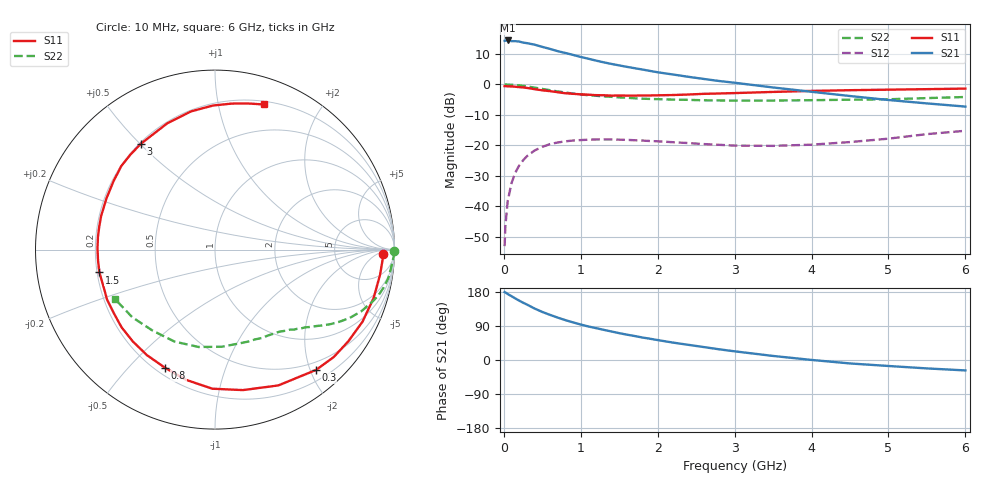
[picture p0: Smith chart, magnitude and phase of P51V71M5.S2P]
! SIEMENS Small Signal Semiconductors
! BFP183
! Si NPN RF Bipolar Junction Transistor in SOT143
! VCE = 1.75 V  IC = 1.5 mA
! Common Emitter S-Parameters:  March  1996
# GHz  S  MA  R  50
!  f  S11  S21  S12  S22
! GHz  MAG  ANG  MAG  ANG  MAG  ANG  MAG  ANG
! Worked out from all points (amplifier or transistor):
!   36 points, 10 MHz to 6 GHz, reference 50 ohm
!   highest |S21| = 14.4 dB at 50 MHz (marker M1)
!   |S21| within 3 dB of that: start of sweep to 630 MHz
!   unconditionally stable (mu >= 1): 2.223 GHz to end of sweep
!   at 250 MHz: K = 0.11, MSG = 19.3 dB, |S12| = -24.9 dB
!   at 1.4 GHz: K = 0.61, MSG = 12.4 dB, |S12| = -18.1 dB
!   at 6 GHz: K = 1.02, MAG = 3.2 dB, |S12| = -15.2 dB
!   S11 on the Smith chart (normalised r, x): 10 MHz: 26, -11; 300 MHz: 0.36, -2.09; 800 MHz: 0.24, -0.64; 1.5 GHz: 0.21, -0.09; 3 GHz: 0.21, +0.50; 6 GHz: 0.23, +1.37
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0.01  0.9373 -1.6  5.195 179.2  0.0022 83.9  0.9994 -0.6
0.02  0.9353 -3.5  5.226 178.3  0.0047 83.9  0.9991 -1.3
0.05  0.9302 -8.8  5.268 174.1  0.0121 86.5  0.993 -3.2
0.1  0.9238 -17.1  5.133 168.4  0.0239 79.3  0.985 -6.4
0.15  0.9148 -26.0  5.126 162.3  0.0358 74.9  0.9778 -9.6
0.2  0.9016 -34.5  5.059 156.6  0.0465 70.0  0.9633 -12.6
0.3  0.8754 -50.0  4.758 146.4  0.0661 61.6  0.9265 -18.0
0.4  0.835 -65.0  4.494 135.8  0.082 53.3  0.8852 -22.8
0.5  0.798 -78.8  4.131 126.8  0.0941 45.8  0.8416 -26.9
0.6  0.7752 -91.1  3.827 119.1  0.1044 40.0  0.8027 -30.0
0.7  0.7437 -102.3  3.511 111.9  0.1111 34.7  0.7665 -32.8
0.8  0.7152 -112.8  3.282 105.2  0.1161 29.9  0.7358 -35.0
0.9  0.6997 -122.8  3.048 99.2  0.1196 25.8  0.7064 -37.1
1.1  0.677 -140.3  2.638 88.4  0.1234 19.0  0.6632 -40.8
1.5  0.6568 -168.8  2.05 70.8  0.1236 9.5  0.6107 -46.9
1.8  0.6561 173.5  1.756 59.4  0.1195 5.4  0.5825 -51.6
2.2  0.6687 154.7  1.452 45.9  0.1122 2.1  0.5623 -58.4
3  0.7199 124.9  1.064 22.9  0.0987 4.2  0.5406 -74.6
3.5  0.7518 110.8  0.89 10.7  0.0977 10.0  0.5424 -85.9
4.5  0.8028 90.8  0.644 -9.1  0.1129 20.6  0.56 -113.8
5.5  0.8348 77.2  0.487 -22.2  0.1524 23.2  0.5954 -140.7
6  0.8532 71.4  0.432 -27.5  0.173 20.1  0.6206 -153.4
